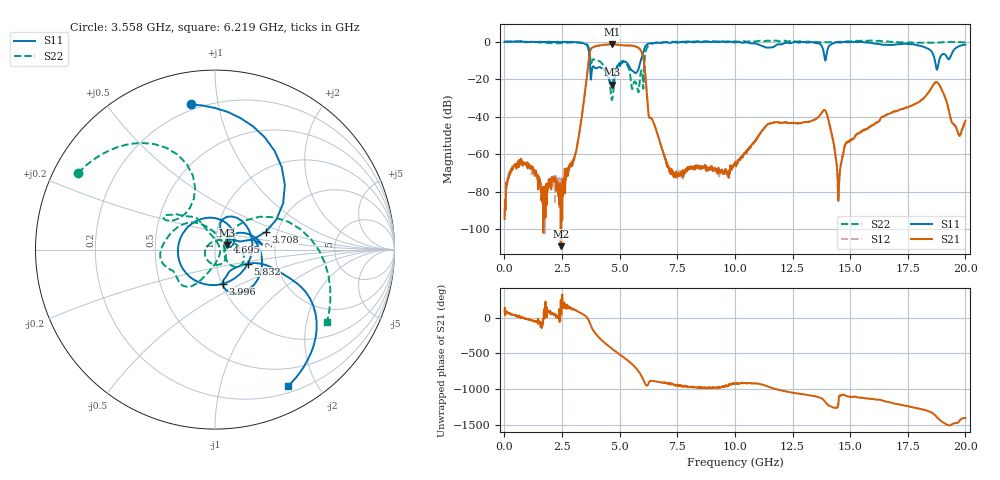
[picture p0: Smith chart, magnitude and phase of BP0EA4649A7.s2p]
! 9/17/2020 12:54:33 PM
! C:\ANRITSUVNA\DATA\MLO\SAMPLES\RAYTHEOM BP\17374_20GH_91720 .S2P
! CHANNEL.1
! TR.MEASUREMENT
! CORRECTED.DATA
# GHZ S RI R 50.0
! FREQ.GHZ  S11RE  S11IM  S31RE  S31IM  S13RE  S13IM  S33RE  S33IM
!; PortSelection: Port_13
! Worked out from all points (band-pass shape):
!   1601 points, 10 MHz to 20 GHz, reference 50 ohm
!   highest |S21| = -1.42 dB at 4.67 GHz (marker M1); lowest = -108.9 dB at 2.446 GHz (marker M2)
!   |S21| within 3 dB of the highest: 3.735 GHz to 5.904 GHz (2.169 GHz wide, 45 % of centre)
!   lowest |S11| = -22.9 dB at 4.658 GHz (marker M3), VSWR 1.15, Z = 57.1 + j2.93 ohm
!   |S11| at or under -10 dB: 3.705 GHz to 5.918 GHz (2.213 GHz wide, 46 % of centre); 13.91835 GHz to 13.93095 GHz (12.6 MHz wide, 0.0905 % of centre); 18.68 GHz to 18.86 GHz (186.2 MHz wide, 0.992 % of centre)
!   |S22| runs from -31.1 to 0.6 dB; largest |S21 - S12| = 0.0019
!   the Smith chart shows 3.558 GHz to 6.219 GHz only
!   S11 on the Smith chart (normalised r, x): 3.558 GHz: 0.17, +0.83; 3.708 GHz: 1.73, +0.37; 3.996 GHz: 1.01, -0.40; 4.695 GHz: 1.14, +0.10; 5.832 GHz: 1.42, -0.23; 6.219 GHz: 0.27, -1.63
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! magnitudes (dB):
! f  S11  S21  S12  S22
! 10 MHz  0.0  -94.5  -93.0  0.0
! 734.6 MHz  0.1  -63.1  -64.2  0.2
! 2.446 GHz  -0.2  -108.9  -78.4  -0.8
! 3.346 GHz  -0.6  -41.0  -41.0  -0.7
! 3.558 GHz  -1.7  -20.8  -20.7  -1.2
! 3.708 GHz  -10.5  -5.7  -5.7  -7.3
! 3.996 GHz  -14.2  -2.4  -2.4  -10.3
! 4.658 GHz  -22.9  -1.4  -1.4  -31.0
! 4.67 GHz  -22.8  -1.4  -1.4  -31.1
! 4.695 GHz  -22.1  -1.4  -1.4  -29.7
! 5.12 GHz  -11.1  -2.0  -2.0  -10.3
! 5.832 GHz  -14.1  -3.4  -3.4  -26.5
! 6.219 GHz  -1.3  -34.4  -34.4  -2.6
! 6.682 GHz  -0.5  -50.6  -50.6  -0.5
! 7.344 GHz  -0.2  -71.2  -70.1  -0.1
! 10.01 GHz  -0.5  -64.8  -64.4  0.2
! 13.34 GHz  -0.3  -42.2  -42.1  -0.3
! 13.95 GHz  -8.8  -37.4  -37.4  -0.3
! 14.52 GHz  -0.5  -74.1  -80.9  -0.1
! 16.68 GHz  -1.8  -38.5  -38.4  0.0
! 18.75 GHz  -14.7  -21.6  -21.5  -0.5
! 20 GHz  -1.6  -42.2  -42.1  -0.4
